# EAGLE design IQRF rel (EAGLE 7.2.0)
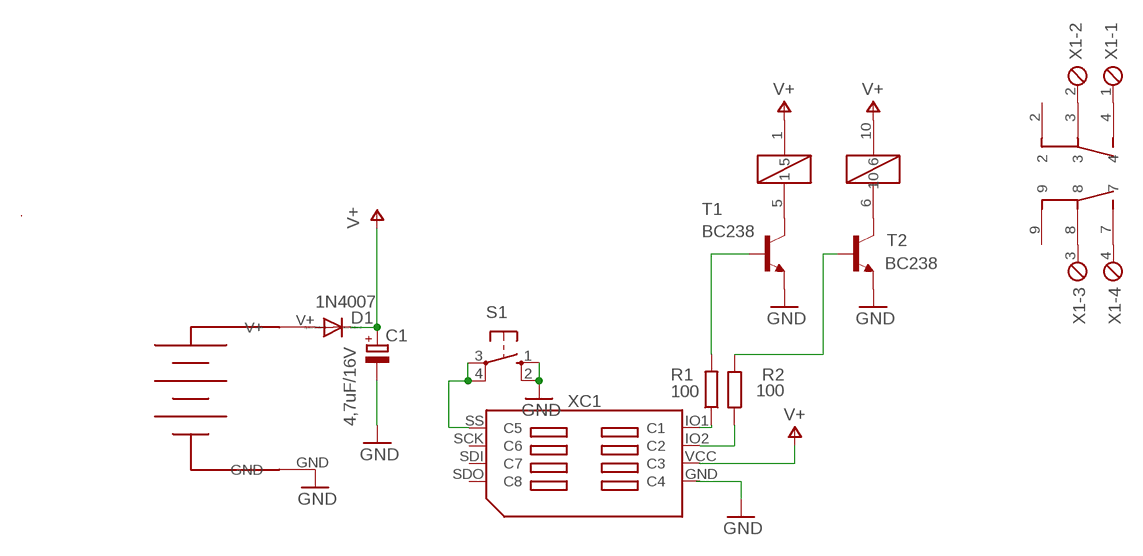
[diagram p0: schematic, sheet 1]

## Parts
C1  4,7uF/16V  CPOL-EUE2,5-6E  [E2,5-6E]
D1  1N4007  DIODE-DO34-7  [DO34-7]
K1  AZ850  [AZ580]
R1  100  R-EU_0207/7  [0207/7]
R2  100  R-EU_0207/7  [0207/7]
S1  10-XX  [B3F-10XX]
T1  BC238  [TO92]
T2  BC238  [TO92]
U$1  3AA  [3AA]
X1  MPT4  [4POL254]
XC1  SIM8X_KON-SIM02  [SIM_02]

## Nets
GND: C1.- S1.1(S) S1.2(S1) T1.1(E) T2.1(E) U$1.GND XC1.GND(C4)
N$1: D1.A U$1.V+
N$2: K1.6 T2.3(C)
N$3: R1.2 T1.2(B)
N$4: R2.1 XC1.IO2(C2)
N$5: R1.1 XC1.IO1(C1)
N$6: K1.4 X1.1
N$7: K1.3 X1.2
N$8: K1.8 X1.3
N$9: K1.7 X1.4
N$11: S1.3(P) S1.4(P1) XC1.SS(C5)
N$12: R2.2 T2.2(B)
N$13: K1.5 T1.3(C)
V+: C1.+ D1.C K1.1 K1.10
Unconnected: K1.2 K1.9 XC1.SCK(C6) XC1.SDI(C7) XC1.SDO(C8) XC1.VCC(C3)

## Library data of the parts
C1 = rcl:CPOL-EU: POLARIZED CAPACITOR, European symbol
D1 = diode:DIODE-: DIODE
K1 = AZ850:AZ850
R1 R2 = rcl:R-EU_: RESISTOR, European symbol
S1 = switch-omron:10-XX: OMRON SWITCH; MPN: B3F-1000; OC_FARNELL: 176432; OC_NEWARK: 36M3542
T1 T2 = transistor:BC238: NPN TRANSISTOR
U$1 = battery:3AA
X1 = con-phoenix-254:MPT4: PHOENIX CONNECTOR; OC_FARNELL: unknown; OC_NEWARK: unknown
XC1 = KON-SIM-02_150624:SIM8X_KON-SIM: KON-SIM-02

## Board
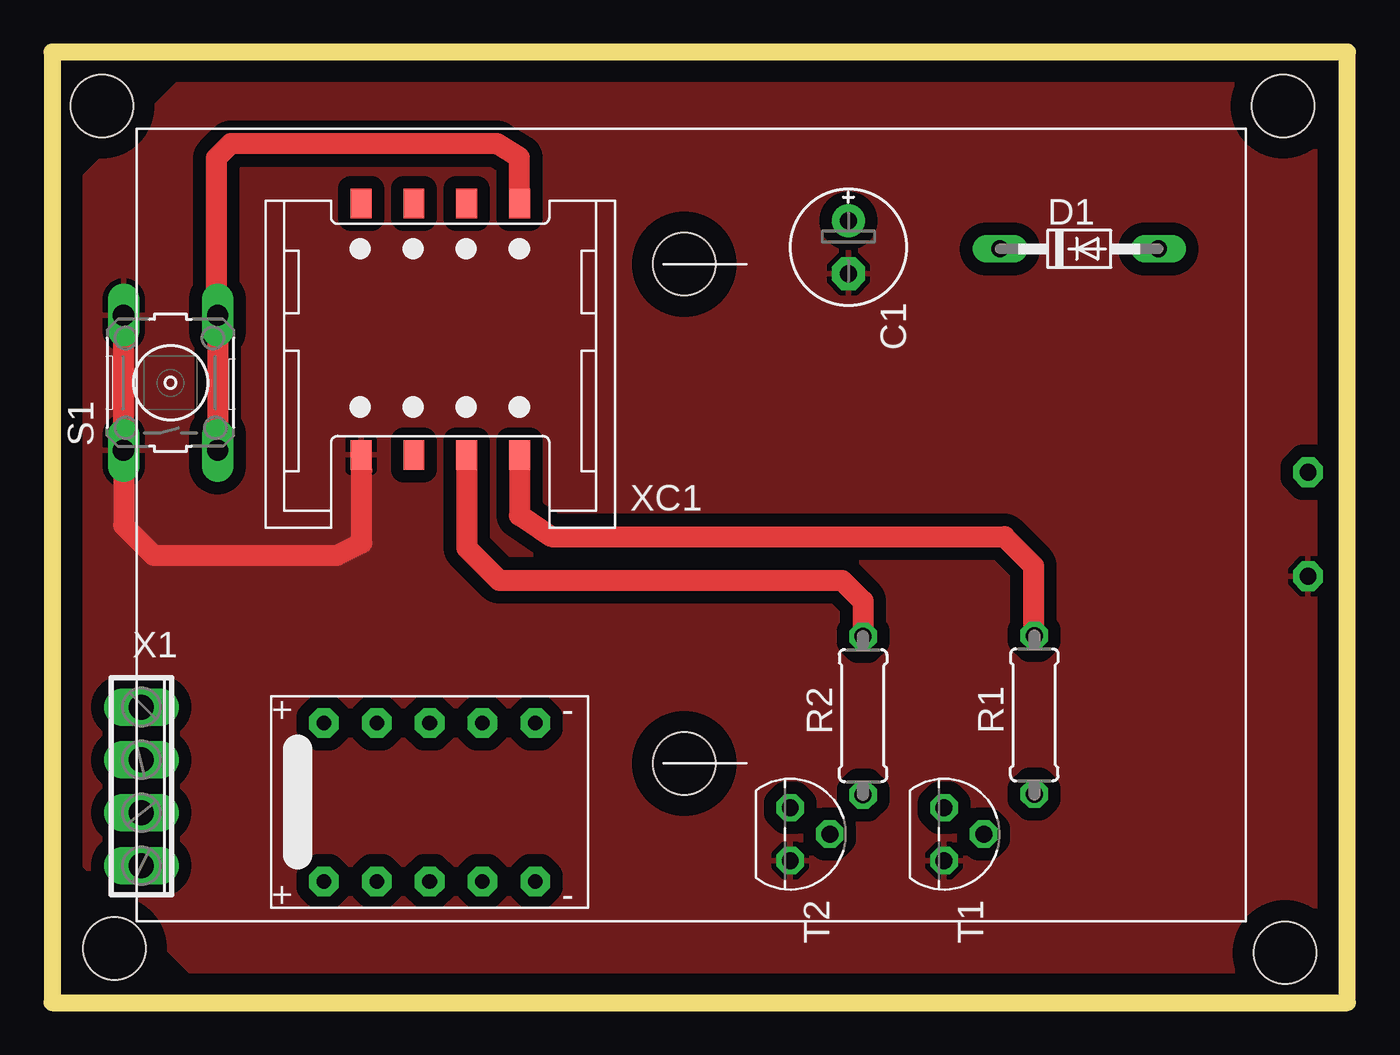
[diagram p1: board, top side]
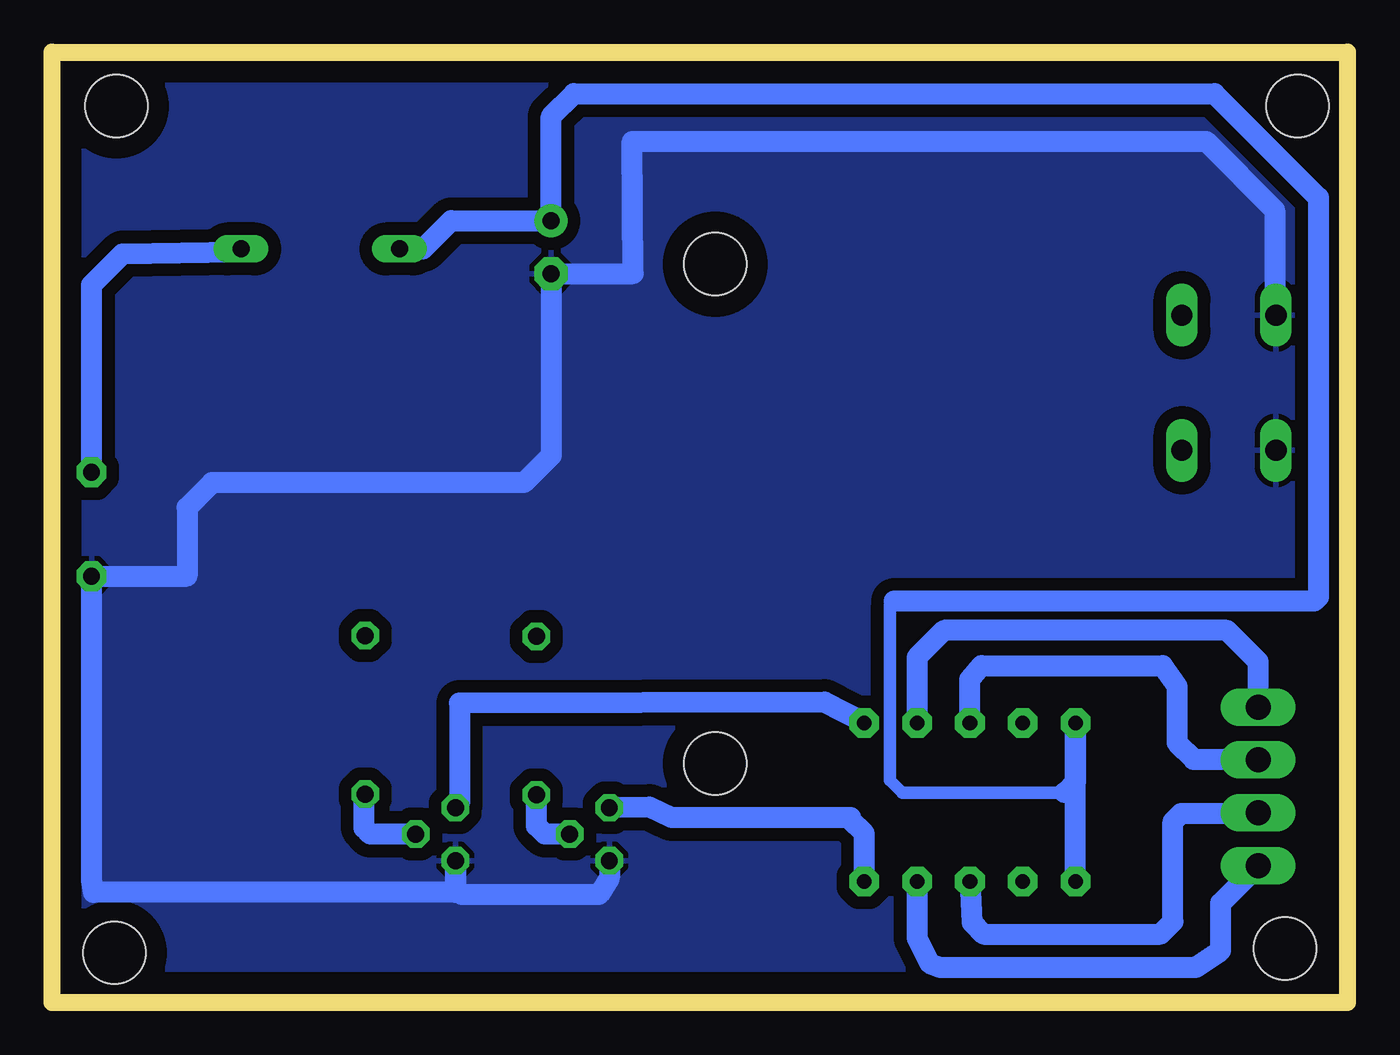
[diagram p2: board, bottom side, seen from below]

Size 62.3 x 45.7 mm. Coordinates in mm from the lower left corner, seen from the top.
Outline: 0,45.7 0,0 62.3,0 62.3,45.7 0,45.7
Copper layers (1*16): Top 0.035mm / dielectric 1.5mm / Bottom 0.035mm
Design rules "default": minimum track width 10mil, minimum drill 24mil, track to track 8mil, track to pad 8mil, pad to pad 8mil, via to via 8mil, smd to smd 8mil, copper to edge 40mil, drill to drill 8mil, minimum pad ring 10mil, minimum via ring 8mil, stop-mask expansion 4mil, vias tented up to drill 0mil, thermal gap 10mil
Holes 3 mm at 2.4,43.1 59.3,2.4 3,2.6 59.2,43.1

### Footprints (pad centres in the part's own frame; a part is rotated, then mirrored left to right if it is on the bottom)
E2,5-6E = drill 0.813 pad 1.575: + -1.27,0 | drill 0.813 pad 1.575 octagon: - 1.27,0
DO34-7 = drill 0.813 long: A 3.81,0; C -3.81,0
AZ580 = drill 0.7 pad 1.422 octagon: 1 -7.62,6.35; 2 -5.08,6.35; 3 -2.54,6.35; 4 0,6.35; 5 2.54,6.35; 6 2.54,-1.27; 7 0,-1.27; 8 -2.54,-1.27; 9 -5.08,-1.27; 10 -7.62,-1.27
0207/7 = drill 0.813 octagon: 1 -3.81,0; 2 3.81,0
B3F-10XX = drill 1.016 long: 1 -3.251,2.261; 2 3.251,2.261; 3 -3.251,-2.261; 4 3.251,-2.261
TO92 = drill 0.813 octagon: 1 1.27,0; 2 0,1.905; 3 -1.27,0
3AA = drill 0.8 pad 1.422 octagon: GND 36,-5; V+ 36,0 | hole 3: 6,10; 6,-14
4POL254 = drill 1.2 long: 1 -3.81,0; 2 -1.27,0; 3 1.27,0; 4 3.81,0
SIM_02 = smd 1.4 x 1: GND 6.112,-3.81; IO1 6.112,3.81; IO2 6.112,1.27; SCK -5.98,1.27; SDI -5.98,-1.27; SDO -5.98,-3.81; SS -5.98,3.81; VCC 6.112,-1.27

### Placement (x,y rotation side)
C1  38.3,36.31 270 top
D1  49.4,36.24 0 top
K1  20.7,7.1 0 top
R1  47.24,13.84 270 top
R2  39,13.8 270 top
S1  5.7,29.8 90 top
T1  42.9,8.1 270 top
T2  35.5,8.1 270 top
U$1  24.4,25.5 0 top
X1  4.3,10.4 270 top
XC1  18.67,32.44 270 top

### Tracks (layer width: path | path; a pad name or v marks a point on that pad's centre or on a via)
GND
  Top 1.016: S1.2 S1.1 3.44,22.96 4.9,21.5 13.7,21.5 14.9,22.1 14.9,25.59 XC1.GND
  Bottom 1.016: T2.1 35.5,6 36,5.2 42.6,5.2 42.9,5.5 T1.1 42.9,5.3 60.3,5.3 60.4,5.9 U$1.GND 55.8,20.5 55.8,23.8 54.6,25 39.6,25 38.3,26.3 C1.- 34.36,35.04 34.4,41.4 6.8,41.4 3.5,38.1 3.5,33.11 S1.2
  pour Top (isolate 0.61): 6.3,44.4 55.8,44.4 62.8,44.6 62.7,1.5 6.7,1.5 0.9,7.3 0.9,39
  pour Bottom (isolate 0.61): 1.1,39.1 6.3,44.4 55.8,44.4 62.8,44.6 62.6,1.6 6.7,1.6 0.9,7.4 0.9,39
N$1
  Bottom 1.016: U$1.V+ 60.4,34.5 58.9,36 53.35,36.1 D1.A
N$2
  Bottom 1.016: T2.3 33.57,9.4 32.5,8.9 23.9,8.9 23.9,8.8 23.24,8.14 K1.6
N$3
  Bottom 1.016: T1.2 47,8.1 47.3,8.4 47.3,9.96 R1.2
N$4
  Top 1.016: XC1.IO2 19.94,21.86 21.5,20.3 38,20.3 39,19.3 R2.1
N$5
  Top 1.016: XC1.IO1 22.48,23.42 24,22.4 45.8,22.4 47.2,21 47.2,17.68 R1.1
N$6
  Bottom 1.016: X1.1 4.3,16.4 5.8,17.9 19.4,17.9 20.7,16.6 20.7,13.55 K1.4
N$7
  Bottom 1.016: K1.3 18.16,15.54 17.6,16.2 8.9,16.2 8.2,15.2 8.2,12.5 7.4,11.7 4.33,11.7 X1.2
N$8
  Bottom 1.016: K1.8 18.06,3.86 17.5,3.3 9,3.3 8.4,3.9 8.4,8.7 8,9.1 4.33,9.1 X1.3
N$9
  Bottom 1.016: K1.7 20.7,3.1 20.1,1.9 19.6,1.7 7.3,1.7 6.1,2.5 6.1,4.79 X1.4
N$11
  Top 1.016: XC1.SS 22.48,40.62 21.4,41.3 8.6,41.3 7.9,40.6 7.9,33.11 S1.4 S1.3
N$12
  Bottom 1.016: T2.2 38.6,8.1 39,8.5 R2.2
N$13
  Bottom 1.016: K1.5 25.15,14.45 42.7,14.4 42.7,9.57 T1.3
V+
  Bottom 0.61: 13.6,10.1 21.4,10.1 22,10.7 22,19.1 21.8,19.3
  Bottom 1.016: K1.10 K1.1 13.08,10.62 13.6,10.1 | D1.C 44.46,36.24 43.1,37.6 38.32,37.6 C1.+ 38.3,42.6 37.2,43.7 6.4,43.7 1.4,38.7 1.4,19.5 1.6,19.3 21.8,19.3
